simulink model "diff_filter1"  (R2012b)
settings: Solver=ode45  StartTime=0.0  StopTime=20  MaxStep=0.001  RelTol=1e-3
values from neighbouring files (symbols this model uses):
  ampl = 1    [diff_filter_1.m]    (also in foerd_gleit_1.m = 0.11; foerder_haft_gleit_1.m = 0.02; foerder_haft_gleit_2.m = 0.02; tilger_gleitreib3.m = 0.01)
  dt = 0.001    [coulomb_1.m]    (also in coulomb_10.m; coulomb_11.m; coulomb_2.m; coulomb_3.m)
  gama = 1e4    (= 10000)    [diff_filter_1.m]    (also in diff_filter_2.m)
  k = 10    [coulomb_10.m]    (also in coulomb_11.m; diff_filter_1.m = 250; diff_filter_2.m = 250; dry_friction_1.m = 2200)
  noise = sqrt(varianz)    [diff_filter_1.m]
  wsig = 2*pi*fsig    (= 6.28318530718)    [diff_filter_1.m]
libraries: dspstat3 x1, simulink x1

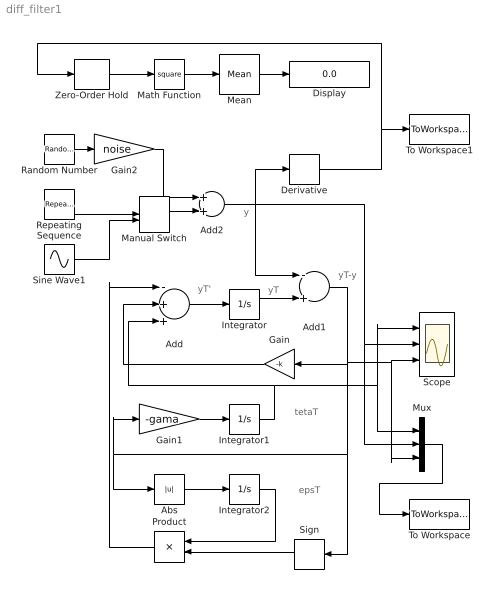
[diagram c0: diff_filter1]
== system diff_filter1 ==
  note: tetaT
  note: epsT
  note: yT-y
  note: y
  note: yT'
  note: yT
  Abs : Abs  ZeroCross=off
  Add : Sum  Inputs=-++
  Add1 : Sum  Inputs=-+
  Add2 : Sum
  Derivative : Derivative
  Display : Display
  Gain : Gain  Gain=-k
  Gain1 : Gain  Gain=-gama
  Gain2 : Gain  Gain=noise
  Integrator : Integrator
  Integrator1 : Integrator
  Integrator2 : Integrator
  Manual Switch : ManualSwitch  CurrentSetting=0
  Math Function : Math  Operator=square
  Mean : dspstat3/Mean  run=on  reset_popup=None  InputProcessing=Columns as channels (frame based)  directionMode=Each column  dimension=1  treatSBRowAsCol=on  roiEnable=off  roiType=Rectangles  roiPortion=Entire ROI  roiOutput=Individual statistics for each ROI  roiFlag=off  outputDataTypeStr=Inherit: Same as accumulator  outputLastDataTypeStr=Inherit: Same as accumulator  outputMin=[]  outputMax=[]  roundingMode=Floor  overflowMode=off
  Mux : Mux  Inputs=3
  Product : Product
  Random Number : RandomNumber  Seed=05793  SampleTime=0
  Repeating Sequence : simulink/Sources/Repeating Sequence  rep_seq_t=tdreieck  rep_seq_y=dreieck
  Scope : Scope  NumInputPorts=3
  Sign : Signum  ZeroCross=off
  Sine Wave1 : Sin  Amplitude=ampl  Frequency=wsig  SampleTime=0
  To Workspace : ToWorkspace  VariableName=y  SampleTime=-1  SaveFormat=Structure With Time
  To Workspace1 : ToWorkspace  VariableName=y1  SampleTime=-1  SaveFormat=Structure With Time
  Zero-Order Hold : ZeroOrderHold  SampleTime=dt
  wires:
  Add/1 -> Integrator/1
  Integrator/1 -> Add1/2
  Gain/1 -> Add/2
  Gain1/1 -> Integrator1/1
  Abs/1 -> Integrator2/1
  Integrator2/1 -> Product/1
  Sign/1 -> Product/2
  Product/1 -> Add/1
  Integrator1/1 -> Add/3, Mux/1, Scope/1
  Random Number/1 -> Gain2/1
  Gain2/1 -> Add2/1
  Add1/1 -> Sign/1, Abs/1, Gain1/1, Mux/3, Scope/3, Gain/1
  Manual Switch/1 -> Add2/2
  Repeating Sequence/1 -> Manual Switch/1
  Sine Wave1/1 -> Manual Switch/2
  Mux/1 -> To Workspace/1
  Mean/1 -> Display/1
  Zero-Order Hold/1 -> Math Function/1
  Math Function/1 -> Mean/1
  Derivative/1 -> To Workspace1/1, Zero-Order Hold/1
  Add2/1 -> Derivative/1, Mux/2, Scope/2, Add1/1
